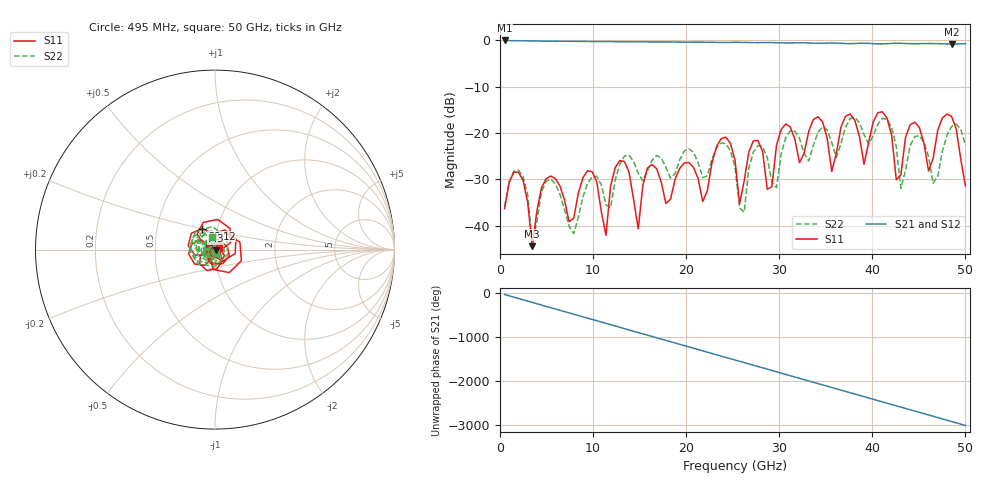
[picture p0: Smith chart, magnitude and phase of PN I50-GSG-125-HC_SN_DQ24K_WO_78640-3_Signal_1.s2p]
!  2-Port S-parameters as saved by WinCal
!VAR DATE=09-27-2011  08:00:25
!VAR OPNAME=Lien Nguyen
# Hz S RI R 50.00
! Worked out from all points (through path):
!   101 points, 495 MHz to 50 GHz, reference 50 ohm
!   highest |S21| = -0.07 dB at 495 MHz (marker M1); lowest = -0.8 dB at 48.51 GHz (marker M2)
!   lowest |S11| = -44.4 dB at 3.465 GHz (marker M3), VSWR 1.01, Z = 50.5 - j0.343 ohm
!   |S11| at or under -10 dB: start of sweep to end of sweep
!   |S22| runs from -43.8 to -16.6 dB; largest |S21 - S12| = 0
!   S11 on the Smith chart (normalised r, x): 495 MHz: 0.99, -0.03; 38.12 GHz: 0.85, +0.20; 50 GHz: 1.05, +0.02
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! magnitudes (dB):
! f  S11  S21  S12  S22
! 495 MHz  -36.3  -0.1  -0.1  -35.9
! 1.98 GHz  -28.5  -0.1  -0.1  -28.0
! 3.465 GHz  -44.4  -0.2  -0.2  -43.8
! 4.95 GHz  -29.9  -0.2  -0.2  -30.5
! 7.426 GHz  -39.2  -0.3  -0.3  -40.1
! 8.911 GHz  -29.7  -0.3  -0.3  -33.8
! 11.39 GHz  -42.1  -0.3  -0.3  -35.5
! 12.87 GHz  -26.0  -0.3  -0.3  -26.8
! 14.85 GHz  -40.7  -0.3  -0.3  -28.7
! 15.84 GHz  -27.6  -0.4  -0.4  -28.2
! 17.33 GHz  -30.7  -0.4  -0.4  -25.4
! 25.25 GHz  -25.8  -0.5  -0.5  -27.3
! 26.24 GHz  -30.3  -0.5  -0.5  -37.1
! 27.72 GHz  -21.7  -0.5  -0.5  -22.8
! 28.71 GHz  -32.2  -0.5  -0.5  -25.3
! 33.66 GHz  -17.1  -0.7  -0.7  -22.7
! 35.64 GHz  -28.3  -0.6  -0.6  -22.1
! 38.12 GHz  -17.3  -0.7  -0.7  -16.6
! 42.08 GHz  -20.6  -0.7  -0.7  -18.8
! 43.07 GHz  -29.0  -0.7  -0.7  -32.0
! 48.51 GHz  -16.4  -0.8  -0.8  -18.6
! 50 GHz  -31.4  -0.7  -0.7  -22.7
